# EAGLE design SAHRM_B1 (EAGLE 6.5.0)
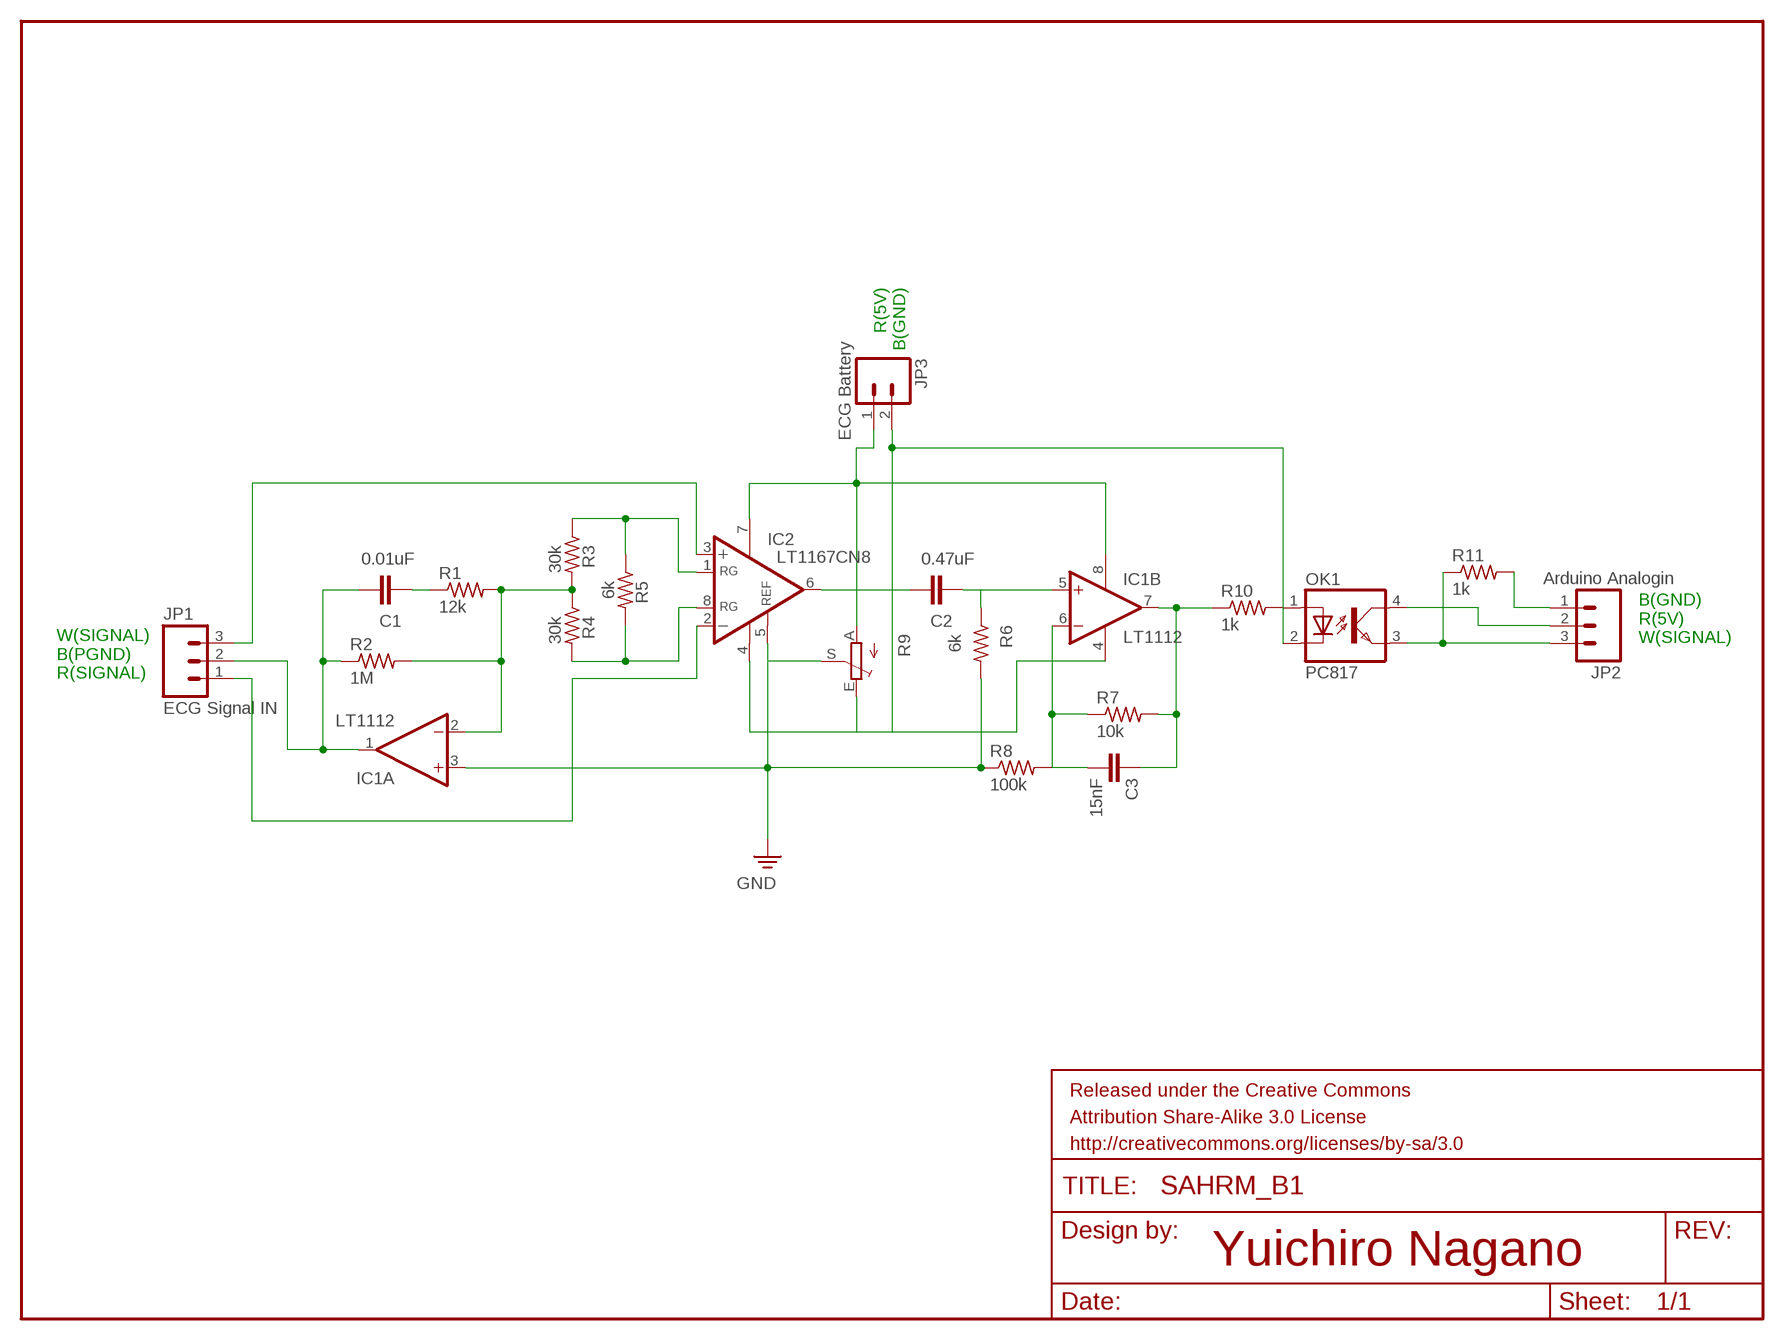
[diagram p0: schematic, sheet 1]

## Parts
C1  0.01uF  C2,5-3  [C2.5-3]
C2  0.47uF  C2,5-3  [C2.5-3]
C3  15nF  C2,5-3  [C2.5-3]
FRAME1  FRAME-LETTER  [CREATIVE_COMMONS]
IC1  LT1112  2AMP_P8+4N  [DIL08]
IC2  LT1167CN8  LT1168CN8  [DIL08]
JP1  ECG Signal IN  M03PTH  [1X03]
JP2  Arduino Analogin  M03PTH  [1X03]
JP3  ECG Battery  M02PTH  [1X02]
OK1  PC817  [DIL04]
R1  12k  R-US_0204/2V  [0204V]
R2  1M  R-US_0204/2V  [0204V]
R3  30k  R-US_0204/2V  [0204V]
R4  30k  R-US_0204/2V  [0204V]
R5  6k  R-US_0204/2V  [0204V]
R6  6k  R-US_0204/2V  [0204V]
R7  10k  R-US_0204/2V  [0204V]
R8  100k  R-US_0204/2V  [0204V]
R9  TRIM_EU-B25P  [B25P]
R10  1k  R-US_0204/2V  [0204V]
R11  1k  R-US_0204/2V  [0204V]

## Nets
B1: IC1.3(A:+IN) IC2.5(REF) R6.2 R8.1 R9.S ; supply symbol labelled GND
N$1: C1.2 IC1.1(A:OUT) JP1.2 R2.1
N$2: IC2.3(+IN) JP1.3
N$3: IC1.2(A:-IN) R1.2 R2.2 R3.2 R4.1
N$4: IC2.1(RG) R3.1 R5.1
N$5: IC2.8(RG) R4.2 R5.2
N$6: IC2.2(-IN) JP1.1
N$7: IC1.8(P:V+) IC2.7(V+) JP3.1 R9.A
N$8: C2.2 IC2.6(OUT)
N$9: C2.1 IC1.5(B:+IN) R6.1
N$10: C3.2 IC1.6(B:-IN) R7.1 R8.2
N$11: C1.1 R1.1
N$12: C3.1 IC1.7(B:OUT) R7.2 R10.1
N$13: IC1.4(P:V-) IC2.4(V-) JP3.2 OK1.2(C) R9.E
N$14: OK1.1(A) R10.2
N$15: JP2.2 OK1.4(COL)
N$16: JP2.3 OK1.3(EMIT) R11.1
N$17: JP2.1 R11.2

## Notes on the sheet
- R(5V)
  B(GND)
- B(GND)
  R(5V)
  W(SIGNAL)
- W(SIGNAL)
  B(PGND)
  R(SIGNAL)
- Yuichiro Nagano

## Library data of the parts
C1-C3 = capacitor-wima:C: CAPACITOR
FRAME1 = SparkFun-Aesthetics:FRAME-LETTER: Schematic Frame
IC1 = linear:2AMP_P8+4: OP AMP
IC2 = linear-technology:LT1168: Low Power, Single Resistor Gain Programmable, Precision Instrumentation Amplifier SourcE: LT1168.pdf; MPN: LT1168CN8#PBF; OC_FARNELL: 1330587; OC_NEWARK: 57M2327
JP1 JP2 = SparkFun-Connectors:M03: Header 3 Standard 3-pin 0.1" header. Use with straight break away headers (SKU : PRT-00116), right angle break away headers (PRT-00553), swiss pins (PRT-00743), machine pins (PRT-00117), and female headers (PRT-00115). Molex polarized connector foot print use with SKU : PRT-08232 with associated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
JP3 = SparkFun-Connectors:M02: Header 2
OK1 = optocoupler:PC817: SHARP OPTO COUPLER; MPN: PC817X4J000F; OC_FARNELL: 9707727; OC_NEWARK: 97K7059
R1-R8 R10 R11 = resistor:R-US_: RESISTOR, American symbol
R9 = pot:TRIM_EU-: POTENTIOMETER

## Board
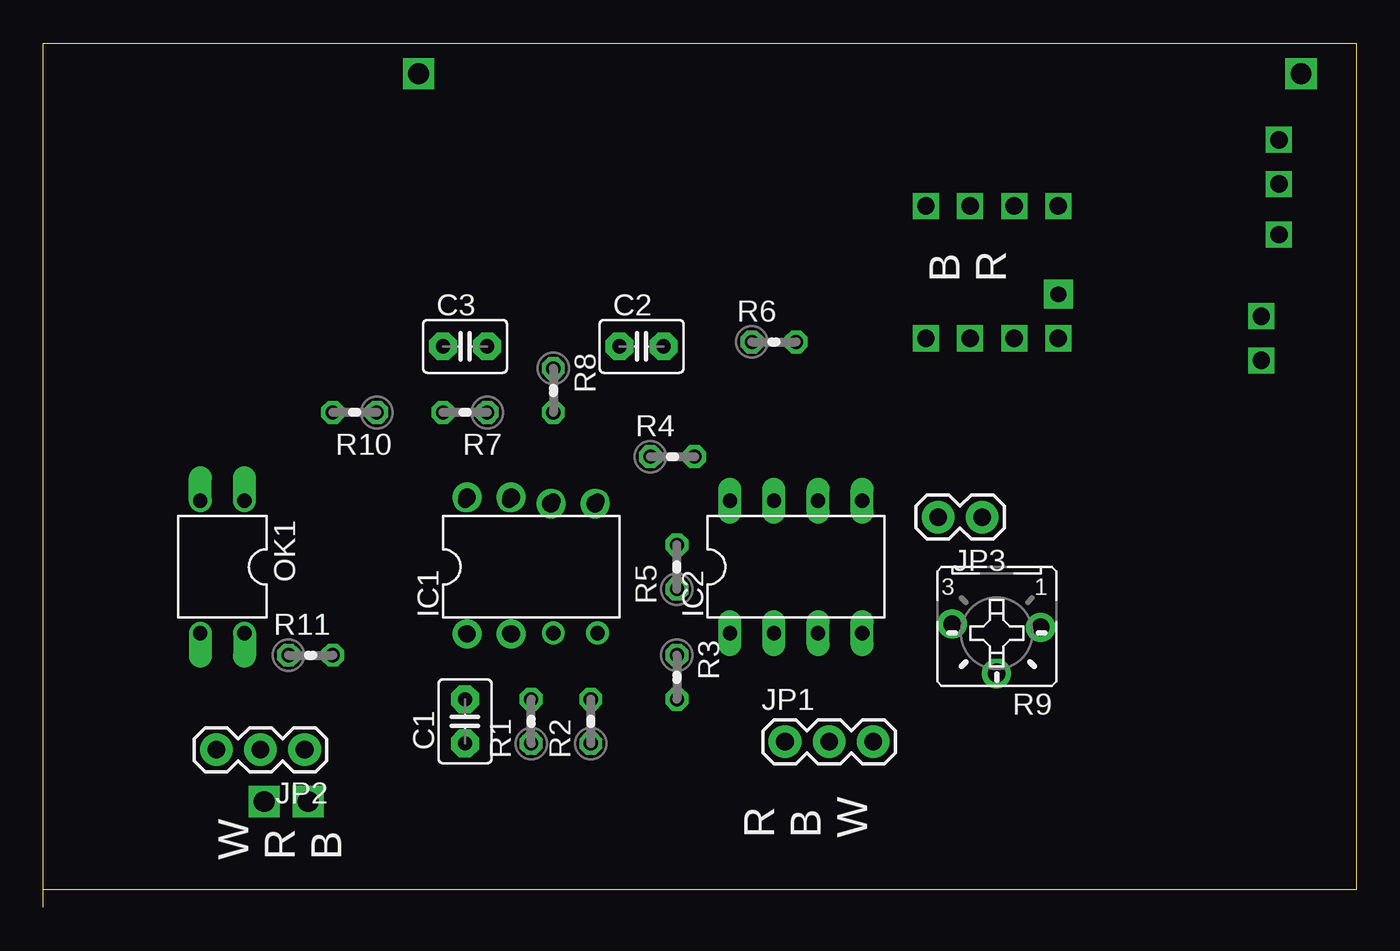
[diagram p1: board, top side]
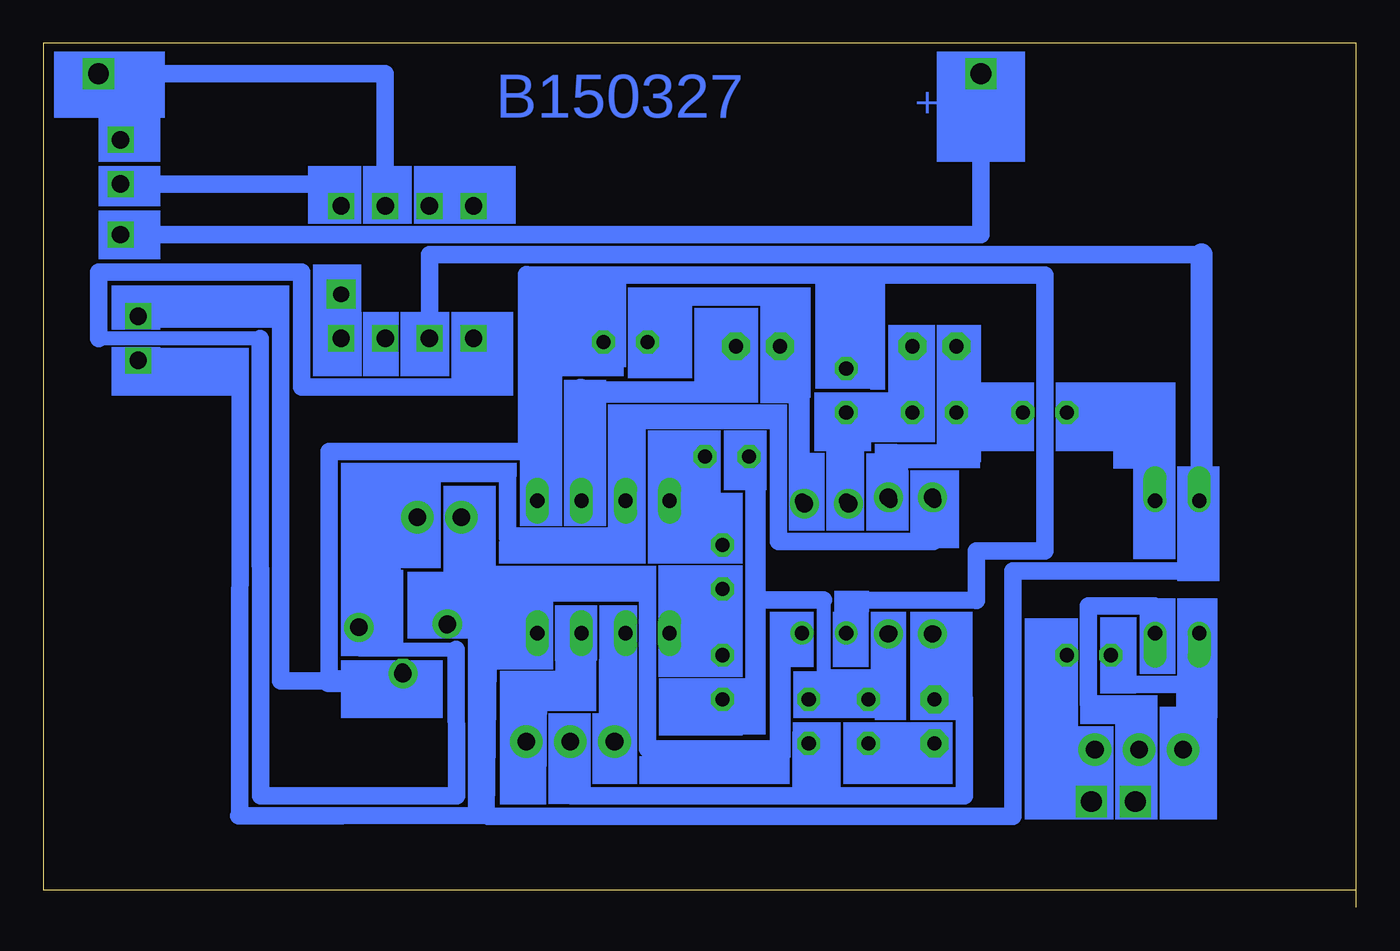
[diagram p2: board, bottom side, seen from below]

Size 75.56 x 49.73 mm. Coordinates in mm from the lower left corner, seen from the top.
Outline: 0,1 75.56,1 75.56,49.73 0,49.73 0,1
Outline: 0,0 0,1
Copper layers (1*16): Top 0.035mm / dielectric 1.5mm / Bottom 0.035mm
Design rules "Fusion_eagle_rule_v1.1": minimum track width 6mil, minimum drill 12mil, track to track 6mil, track to pad 6mil, pad to pad 6mil, via to via 6mil, smd to smd 0mil, copper to edge 10mil, drill to drill 10mil, minimum pad ring 10mil, minimum via ring 6mil, stop-mask expansion 2mil, vias tented up to drill 100mil, thermal gap 10mil

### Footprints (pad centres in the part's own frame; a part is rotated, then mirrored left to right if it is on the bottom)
C2.5-3 = drill 0.813 pad 1.6 octagon: 1 -1.27,0; 2 1.27,0
DIL08 = drill 0.813 pad 1.27: 1 -3.81,-3.81; 2 -1.27,-3.81; 3 1.27,-3.81; 4 3.81,-3.81; 5 3.81,3.81; 6 1.27,3.81; 7 -1.27,3.81; 8 -3.81,3.81
DIL08' = drill 0.813 long: 1 -3.81,-3.81; 2 -1.27,-3.81; 3 1.27,-3.81; 4 3.81,-3.81; 5 3.81,3.81; 6 1.27,3.81; 7 -1.27,3.81; 8 -3.81,3.81
1X03 = drill 1.016 pad 1.88: 1 0,0; 2 2.54,0; 3 5.08,0
1X02 = drill 1.016 pad 1.88: 1 0,0; 2 2.54,0
DIL04 = drill 0.813 offset: 1 -1.27,-3.81; 2 1.27,-3.81; 3 1.27,3.81; 4 -1.27,3.81
0204V = drill 0.813 octagon: 1 -1.27,0; 2 1.27,0
B25P = drill 0.813 octagon: A -2.54,0; E 2.54,0; S 0,2.54

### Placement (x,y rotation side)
C1  24.27,10.7 90 top
C2  34.43,32.29 0 top
C3  24.27,32.29 0 top
FRAME1  not placed on the board
IC1  28.08,19.59 0 top
IC2  LT1167CN8  [DIL08']  43.32,19.59 0 top
JP1  42.69,9.52 0 top
JP2  15.03,9.07 180 top
JP3  54.04,22.46 180 top
OK1  10.3,19.59 180 top
R1  28.08,10.7 90 top
R2  31.51,10.7 90 top
R3  36.46,13.24 270 top
R4  36.21,25.94 0 top
R5  36.46,19.59 90 top
R6  42.05,32.54 0 top
R7  24.27,28.48 180 top
R8  29.35,29.75 270 top
R9  54.88,16.16 180 top
R10  17.92,28.48 180 top
R11  15.38,14.51 0 top

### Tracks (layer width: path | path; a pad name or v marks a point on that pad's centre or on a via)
B1
  Bottom 0.254: 47.18,23.94 IC2.5 | 54.93,13.02 R9.S | 43.37,31.56 R6.2 | 29.15,31.05 R8.1
  Bottom 1.016: 29.15,36.39 17.92,36.39 17.92,20.51 21.84,20.51 21.84,17.66 29.35,17.69 IC1.3 | 70.04,34.1 68.77,34.02 61.9,34.02 61.91,13.02 59.12,13.02 59.12,26.23 47.75,26.23 47.75,36.43 43.37,36.39 | 47.18,23.94 46.35,23.94 46.35,26.15 46.42,31.56 43.37,31.56 43.37,36.39 | 29.15,36.39 29.15,31.05 | 43.37,36.39 29.15,36.39
  Bottom 1.27: 59.12,13.02 54.93,13.02
N$1
  Bottom 0.254: 24.32,16.32 IC1.1 | 24.32,12.51 C1.2 24.32,12 | 31.94,9.97 R2.1
  Bottom 0.61: 45.15,7.94 JP1.2
  Bottom 1.016: 31.94,6.41 45.15,6.41 45.15,7.94 | 24.32,12 22.54,12 22.54,6.41 31.94,6.41 | 31.94,9.97 31.94,6.41
  Bottom 1.27: 24.32,12.51 24.32,16.32
N$2
  Bottom 0.254: 44.64,15.05 IC2.3
  Bottom 1.27: 44.64,15.05 44.64,12.51 47.69,12.51 JP1.3
N$3
  Bottom 0.254: 31.94,12.51 R2.2 | 26.86,16.32 IC1.2 | 26.86,12.26 R1.2 | 34.48,25.21 R4.1
  Bottom 0.61: 30.67,12.51 31.94,12.51
  Bottom 0.813: 30.67,17.69 30.67,12.51
  Bottom 1.016: 34.48,17.69 34.48,11.95 R3.2 | 34.48,25.21 34.48,17.69 | 34.48,17.69 30.67,17.69
  Bottom 1.27: 30.67,12.51 26.86,12.26 26.86,16.32
N$4
  Bottom 0.254: 39.56,16.32 IC2.1 | 36.26,18.86 R5.1
  Bottom 0.406: 39.31,16.32 39.56,16.32
  Bottom 0.813: 36.26,18.86 36.26,16.32 R3.1
  Bottom 1.016: 39.31,16.32 36.26,16.32
N$5
  Bottom 0.254: 36.26,21.4 R5.2 | 37.27,25.97 R4.2
  Bottom 0.406: 36.77,25.97 37.27,25.97 37.53,25.97
  Bottom 0.61: 37.53,21.4 36.26,21.4 | 39.56,22.67 IC2.8
  Bottom 1.27: 39.56,22.67 39.56,21.4 37.53,21.4 37.53,25.97
N$6
  Bottom 0.254: 42.1,15.05 IC2.2 | 42.1,9.46 JP1.1
  Bottom 1.016: 42.1,9.46 42.1,15.05
N$7
  Bottom 0.254: 54.8,24.96 JP3.1 | 24.32,23.94 IC1.8
  Bottom 0.61: 42.1,22.67 IC2.7 42.1,23.94
  Bottom 0.813: 54.8,21.4 57.47,21.4 R9.A | 24.32,21.04 24.32,23.94
  Bottom 1.016: 54.8,24.96 54.8,21.4 | 42.1,22.67 42.1,21.27 48.85,21.27 48.85,24.96 54.55,24.96 JP3.1 | 24.32,21.04 33.26,21.04 33.26,28.26 42.1,28.26
  Bottom 1.27: 42.1,23.94 42.1,28.26
N$8
  Bottom 0.254: 44.64,23.94 IC2.6
  Bottom 1.016: 44.64,29.78 35.75,29.78 C2.2
  Bottom 1.27: 44.64,29.78 44.64,23.94
N$9
  Bottom 0.254: 31.94,23.94 IC1.5 | 33.21,31.56 C2.1
  Bottom 0.813: 31.94,29.53 33.21,29.53 C2.1 | 33.21,31.56 33.21,35.12 | 40.83,35.12 R6.1
  Bottom 1.016: 31.94,29.53 31.94,23.94 | 33.21,35.12 40.83,35.12
N$10
  Bottom 0.254: 25.59,31.56 C3.2 | 25.59,28.51 R7.1
  Bottom 0.61: 29.4,28.26 R8.2 | 29.4,23.94 IC1.6
  Bottom 1.016: 25.59,31.56 25.59,28.51 29.4,28.26 29.4,23.94
N$11
  Bottom 0.254: 28.13,9.46 R1.1 | 24.32,9.46 C1.1
  Bottom 0.61: 24.32,9.46 28.13,9.46
N$12
  Bottom 0.254: 23.05,27.75 23.05,29.02 R7.2 | 26.86,23.94 IC1.7 | 19.24,29.02 R10.1 | 23.05,31.56 C3.1
  Bottom 1.016: 23.05,27.75 23.05,26.15 26.92,26.15 26.86,23.94 | 19.24,29.02 23.05,29.02 23.05,31.56
N$13
  Bottom 0.254: 31.94,15.56 IC1.4 | 47.18,15.81 IC2.4 | 50.99,18.1 R9.E
  Bottom 0.61: 33.21,15.56 31.94,15.56 | 50.99,22.42 JP3.2
  Bottom 1.016: 50.08,5.29 64.31,5.27 58.38,5.27 | 33.21,15.56 33.21,9.11 40.78,9.11 40.78,18.1 47.18,18.1 | 47.18,18.1 47.18,15.81 49.97,14.03 50.08,5.29 | 47.18,18.1 50.99,18.1 | 50.99,18.1 52.2,18.1 52.2,16.24 50.99,18.1 | 50.08,5.29 49.97,5.25 19.75,5.25 19.75,19.37 9.08,19.37 OK1.2 | 50.99,18.1 50.99,22.42
N$14
  Bottom 0.254: 11.62,23.94 OK1.1
  Bottom 0.61: 16.7,28.51 R10.2
  Bottom 1.016: 11.62,23.94 11.62,28.51 16.7,28.51
N$15
  Bottom 0.254: 11.89,8.7 12.61,8
  Bottom 0.61: 11.62,17.34 OK1.4
  Bottom 0.813: 12.34,11.72 15.4,11.72
  Bottom 1.016: 11.62,17.34 15.4,17.34 15.4,11.72 | 12.34,11.72 JP2.2
N$16
  Bottom 0.254: 9.84,8.19 JP2.3 | 9.08,15.05 OK1.3
  Bottom 1.016: 9.87,12.81 14.06,12.81 R11.1 | 9.84,8.19 9.87,12.81 | 9.87,12.81 9.14,12 9.14,12.81 9.08,15.05
N$17
  Bottom 0.254: 15.43,7.94 JP2.1
  Bottom 0.61: 17.97,15.05 R11.2
  Bottom 1.016: 17.97,15.05 17.97,7.94 15.43,7.94
N$18  (via drill 1 pad 1.68)
  other vias: 52.31,16.3
N$19  (via drill 1 pad 1.68)
  other vias: 54.86,13.45
N$20  (via drill 1 pad 1.68)
  other vias: 57.4,16.11
N$21  (via drill 1 pad 1.68)
  other vias: 31.75,23.23
N$22  (via drill 1 pad 1.68)
  other vias: 29.21,23.23
N$23  (via drill 1 pad 1.68)
  other vias: 24.38,23.61
N$24  (via drill 1 pad 1.68)
  other vias: 26.92,23.61
N$25  (via drill 1 pad 1.68)
  other vias: 24.38,15.73
N$26  (via drill 1 pad 1.68)
  other vias: 26.92,15.73
N$27  (via drill 1 pad 1.27)
  other vias: 70.1,31.48
N$28  (via drill 1 pad 1.27)
  other vias: 70.1,34.02
N$29
  Bottom 1.016: 64.26,5.39 64.24,31.53 71.12,31.48
N$30  (via drill 1 pad 1.27)
  Bottom 1.016: v58.42,40.37 58.42,41.64 v71.12,41.64
N$31  (via drill 1 pad 1.27, 1.2 pad 1.68)
  Bottom 0.61: v71.12,44.18 v72.39,47.99 71.88,47.99
  Bottom 1.016: v55.88,40.37 55.88,47.99 71.88,47.99
N$32  (via drill 1 pad 1.27)
  Bottom 0.813: 57.4,16.24 57.4,14.84 51.82,14.84 | 63.09,32.75 72.39,32.75
  Bottom 1.016: 63.09,32.75 63.07,6.41 51.79,6.41 51.82,14.84 | 72.39,32.75 72.39,36.56 60.71,36.56 60.71,29.96 50.8,29.96 v50.8,32.75
N$33  (via drill 1 pad 1.27)
  Bottom 0.61: v50.8,40.37 v53.34,40.37
N$34  (via drill 1 pad 1.27)
  Bottom 1.016: 26.67,38.72 v71.12,38.72
N$35  (via drill 1 pad 1.27)
  Bottom 1.016: 8.89,37.58 53.34,37.58 v53.34,32.75
  Bottom 1.27: 8.89,25.13 8.89,37.58
N$36  (via drill 0.9 pad 1.68)
  other vias: 58.42,35.29
N$37  (via drill 1 pad 1.27)
  other vias: 55.88,32.75
N$38  (via drill 1 pad 1.27)
  other vias: 58.42,32.75
N$39  (via drill 1.2 pad 1.68)
  other vias: 12.7,6.08
N$40  (via drill 1.2 pad 1.68)
  other vias: 15.24,6.08
N$64  (via drill 1.2 pad 1.68)
  Bottom 1.016: 26.67,38.72 21.59,38.72 v21.59,47.99
(copper drawn outside any net)
  shapes: Bottom area x232

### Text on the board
Bottom: - | + | B150327
tPlace: B / R | R / B / W | W / R / B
